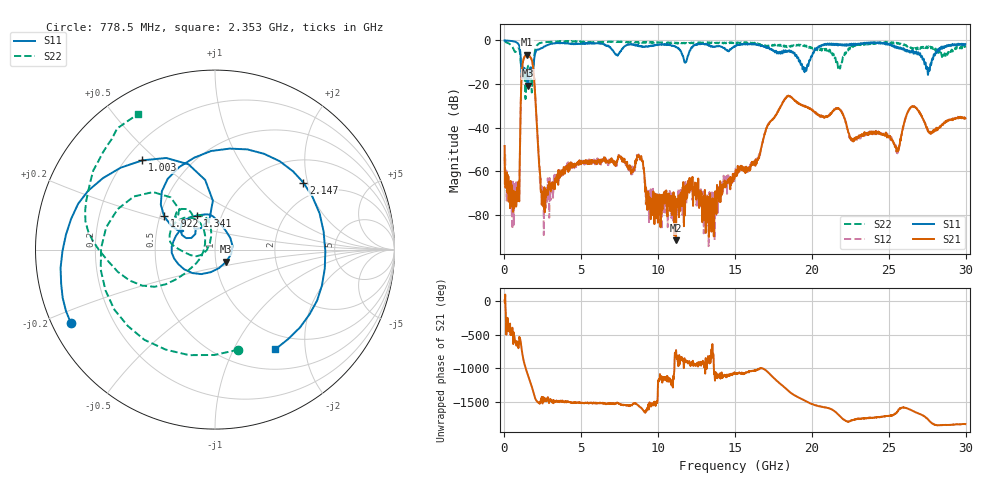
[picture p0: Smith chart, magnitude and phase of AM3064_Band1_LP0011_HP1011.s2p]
# Hz S DB R 50.0
!freq dBS11 angS11 dBS21 angS21 dBS12 angS12 dBS22 angS22
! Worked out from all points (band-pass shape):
!   1600 points, 10 MHz to 29.98 GHz, reference 50 ohm
!   highest |S21| = -6.50 dB at 1.453 GHz (marker M1); lowest = -91.6 dB at 11.16 GHz (marker M2)
!   |S21| within 3 dB of the highest: 1.212 GHz to 1.796 GHz (583.9 MHz wide, 38.8 % of centre)
!   lowest |S11| = -20.7 dB at 1.547 GHz (marker M3), VSWR 1.20, Z = 56.1 - j7.66 ohm
!   |S11| at or under -10 dB: 1.071 GHz to 1.915 GHz (844.2 MHz wide, 56.5 % of centre); 19.24 GHz to 19.81 GHz (561.1 MHz wide, 2.87 % of centre); 27.3 GHz to 27.78 GHz (481.1 MHz wide, 1.75 % of centre)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
!   |S22| runs from -26.8 to -0.3 dB; largest |S21 - S12| = 0.0057
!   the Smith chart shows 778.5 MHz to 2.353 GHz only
!   S11 on the Smith chart (normalised r, x): 778.5 MHz: 0.05, -0.24; 1.003 GHz: 0.27, +0.45; 1.341 GHz: 0.77, +0.30; 1.922 GHz: 0.53, +0.22; 2.147 GHz: 1.56, +1.88; 2.353 GHz: 0.77, -1.48
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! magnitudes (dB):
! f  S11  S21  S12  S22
! 10 MHz  0.0  -48.3  -53.4  -0.3
! 778.5 MHz  -0.9  -75.1  -69.7  -4.8
! 1.003 GHz  -3.9  -51.6  -51.1  -5.3
! 1.172 GHz  -16.2  -11.3  -11.2  -11.9
! 1.341 GHz  -13.4  -7.1  -7.1  -21.6
! 1.453 GHz  -17.0  -6.5  -6.5  -15.5
! 1.547 GHz  -20.7  -6.7  -6.6  -11.7
! 1.922 GHz  -9.4  -16.6  -16.6  -8.1
! 2.147 GHz  -4.2  -42.7  -42.7  -2.0
! 2.353 GHz  -3.8  -68.1  -63.2  -1.2
! 5.015 GHz  -1.5  -55.7  -55.8  -0.6
! 8.763 GHz  -2.7  -53.1  -53.5  -1.1
! 10 GHz  -2.0  -73.4  -77.2  -0.9
! 11.16 GHz  -3.1  -91.6  -78.6  -1.2
! 15 GHz  -2.7  -61.6  -61.6  -1.3
! 18.34 GHz  -5.3  -25.9  -25.8  -2.6
! 19.99 GHz  -7.5  -31.8  -31.8  -3.4
! 25 GHz  -1.6  -44.3  -43.7  -1.1
! 25.61 GHz  -3.2  -50.6  -50.6  -1.3
! 26.55 GHz  -4.6  -30.3  -30.0  -4.2
! 27.56 GHz  -15.1  -41.7  -41.5  -2.9
! 29.98 GHz  -1.7  -35.7  -35.6  -3.3
